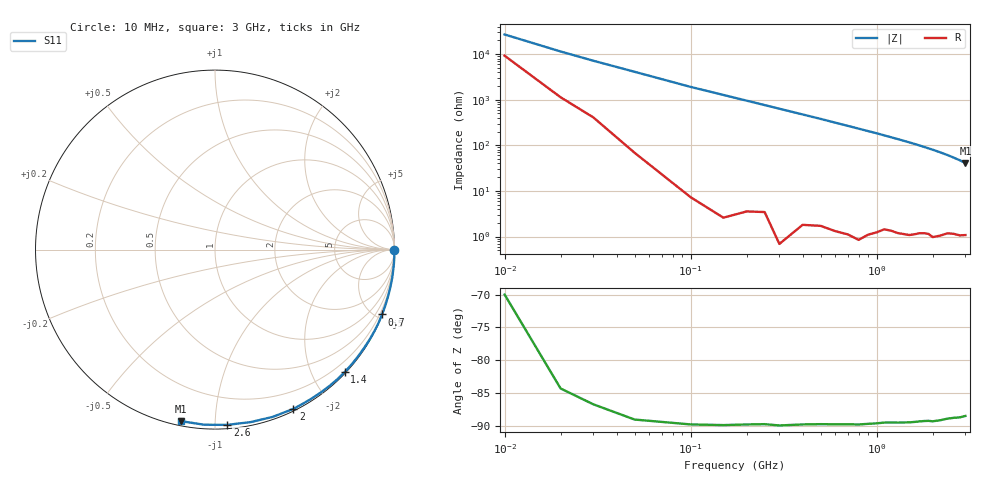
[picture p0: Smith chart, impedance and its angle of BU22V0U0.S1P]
! SIEMENS Small Signal Semiconductors
! BB833
! Si Tuning Diode in SOD323
! VR = 22 V
! S-Parameters:  April  1996
# GHz  S  MA  R  50
!  f  S11
! GHz  MAG  ANG
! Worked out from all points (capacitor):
!   31 points, 10 MHz to 3 GHz, reference 50 ohm
!   read as one part to ground: C = 701 fF near 10 MHz
!   lowest |Z| = 41 ohm at 3 GHz (marker M1)
!   S11 on the Smith chart (normalised r, x): 10 MHz: open; 700 MHz: 0.02, -5.34; 1.4 GHz: 0.02, -2.51; 2 GHz: 0.02, -1.61; 2.6 GHz: 0.02, -1.07; 3 GHz: 0.02, -0.82
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0.01  0.9987 -0.2
0.05  0.9996 -1.4
0.1  0.9998 -3.0
0.15  0.9998 -4.5
0.2  0.9996 -6.0
0.3  0.9998 -9.0
0.4  0.9992 -12.0
0.5  0.9988 -15.0
0.6  0.9987 -18.1
0.7  0.9985 -21.2
0.8  0.9985 -24.3
0.9  0.9975 -27.4
1  0.9966 -30.4
1.1  0.9951 -33.7
1.2  0.9947 -36.9
1.3  0.9944 -40.1
1.4  0.9938 -43.4
1.5  0.9932 -46.6
1.6  0.992 -50.0
1.7  0.9905 -53.4
1.8  0.9893 -56.9
1.9  0.9885 -60.4
2  0.9892 -63.8
2.2  0.9859 -71.0
2.4  0.9814 -78.3
2.6  0.9789 -86.0
2.8  0.9777 -93.5
3  0.9745 -101.3
